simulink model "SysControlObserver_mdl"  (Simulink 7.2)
settings: Solver=ode45  StartTime=0.0  StopTime=10.0  RelTol=1e-3
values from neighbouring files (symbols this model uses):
  A = [ -b1/Ma  -K   b1/Mr         0    [Esercitazione05.m]
  B = [1    [Esercitazione05.m]
  Bd = [-Ma    0    [Esercitazione05.m]
  C = [1/Ma  0   0  0]    [Esercitazione05.m]
  g = 9.81    [Esercitazione05.m]
  Kcontr = -acker(A,B,P)    [Esercitazione05.m]
  L = - acker(A',C',Po)'    [Esercitazione05.m]
  X0 = [0 0.05 0 0]'    [Esercitazione05.m]

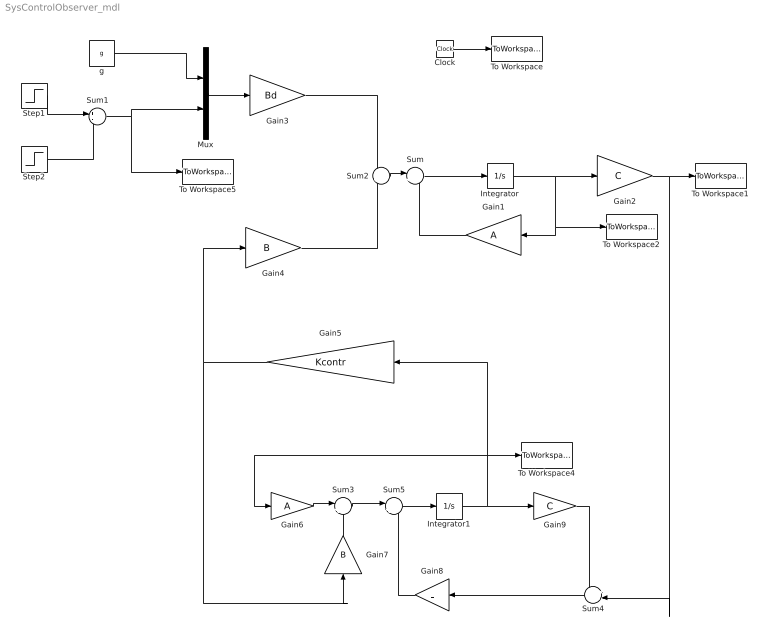
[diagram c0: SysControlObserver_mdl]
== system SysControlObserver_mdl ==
  Clock : Clock
  Gain1 : Gain  Orientation=left  Gain=A  Multiplication=Matrix(K*u)  ParameterDataType=sfix(16)  ParameterScaling=2^0  OutDataType=sfix(16)  OutScaling=2^0
  Gain2 : Gain  Gain=C  Multiplication=Matrix(K*u)  ParameterDataType=sfix(16)  ParameterScaling=2^0  OutDataType=sfix(16)  OutScaling=2^0
  Gain3 : Gain  Gain=Bd  Multiplication=Matrix(K*u)  ParameterDataType=sfix(16)  ParameterScaling=2^0  OutDataType=sfix(16)  OutScaling=2^0
  Gain4 : Gain  Gain=B  Multiplication=Matrix(K*u)  ParameterDataType=sfix(16)  ParameterScaling=2^0  OutDataType=sfix(16)  OutScaling=2^0
  Gain5 : Gain  Orientation=left  Gain=Kcontr  Multiplication=Matrix(K*u)  ParameterDataType=sfix(16)  ParameterScaling=2^0  OutDataType=sfix(16)  OutScaling=2^0
  Gain6 : Gain  Gain=A  Multiplication=Matrix(K*u)  ParameterDataType=sfix(16)  ParameterScaling=2^0  OutDataType=sfix(16)  OutScaling=2^0
  Gain7 : Gain  Orientation=up  Gain=B  Multiplication=Matrix(K*u)  ParameterDataType=sfix(16)  ParameterScaling=2^0  OutDataType=sfix(16)  OutScaling=2^0
  Gain8 : Gain  Orientation=left  Gain=L  Multiplication=Matrix(K*u)  ParameterDataType=sfix(16)  ParameterScaling=2^0  OutDataType=sfix(16)  OutScaling=2^0
  Gain9 : Gain  Gain=C  Multiplication=Matrix(K*u)  ParameterDataType=sfix(16)  ParameterScaling=2^0  OutDataType=sfix(16)  OutScaling=2^0
  Integrator : Integrator  InitialCondition=X0
  Integrator1 : Integrator  InitialCondition=[0 0 0 0]
  Mux : Mux  Inputs=2
  Step1 : Step  Time=5  SampleTime=0
  Step2 : Step  Time=5+0.2  SampleTime=0
  Sum : Sum  Inputs=|++  OutDataType=sfix(16)  OutScaling=2^0
  Sum1 : Sum  Inputs=+-  OutDataType=sfix(16)  OutScaling=2^0
  Sum2 : Sum  OutDataType=sfix(16)  OutScaling=2^0
  Sum3 : Sum  Inputs=|++  OutDataType=sfix(16)  OutScaling=2^0
  Sum4 : Sum  Orientation=left  Inputs=+-  OutDataType=sfix(16)  OutScaling=2^0
  Sum5 : Sum  Inputs=|++  OutDataType=sfix(16)  OutScaling=2^0
  To Workspace : ToWorkspace  VariableName=time  SampleTime=-1  SaveFormat=Array
  To Workspace1 : ToWorkspace  VariableName=y  SampleTime=-1  SaveFormat=Array
  To Workspace2 : ToWorkspace  VariableName=X  SampleTime=-1  SaveFormat=Array
  To Workspace4 : ToWorkspace  VariableName=Xo  SampleTime=-1  SaveFormat=Array
  To Workspace5 : ToWorkspace  VariableName=dXs  SampleTime=-1  SaveFormat=Array
  g : Constant  Value=g  OutDataType=sfix(16)  OutScaling=2^0
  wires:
  Gain1/1 -> Sum/2
  Sum/1 -> Integrator/1
  Integrator/1 -> Gain2/1, To Workspace2/1, Gain1/1
  Clock/1 -> To Workspace/1
  Gain2/1 -> To Workspace1/1, Sum4/2
  Mux/1 -> Gain3/1
  g/1 -> Mux/1
  Step1/1 -> Sum1/1
  Step2/1 -> Sum1/2
  Sum2/1 -> Sum/1
  Sum1/1 -> Mux/2, To Workspace5/1
  Gain3/1 -> Sum2/1
  Gain4/1 -> Sum2/2
  Gain5/1 -> Gain4/1, Gain7/1
  Gain6/1 -> Sum3/1
  Integrator1/1 -> Gain9/1, Gain6/1, To Workspace4/1, Gain5/1
  Gain7/1 -> Sum3/2
  Sum4/1 -> Gain8/1
  Gain9/1 -> Sum4/1
  Gain8/1 -> Sum5/2
  Sum3/1 -> Sum5/1
  Sum5/1 -> Integrator1/1
